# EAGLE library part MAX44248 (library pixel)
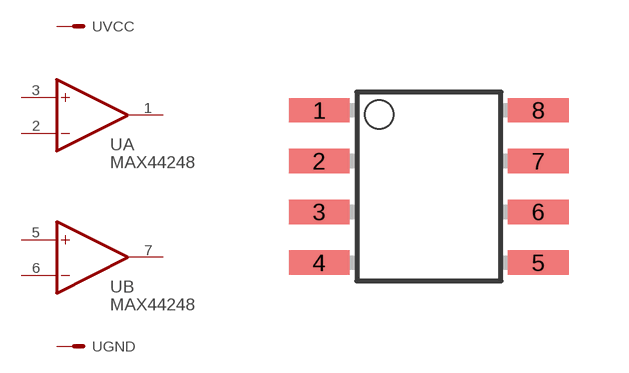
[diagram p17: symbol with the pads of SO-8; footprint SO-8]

Designator prefix -; gates A=OPAMP B=OPAMP VCC=M GND=M

## MAX44248  [SO-8]
1  A:OUT  out
2  A:-IN  in
3  A:+IN  in
4  GND:S  pas
5  B:+IN  in
6  B:-IN  in
7  B:OUT  out
8  VCC:S  pas

## Footprint SO-8 (pad centres in mm)
SO 8 small outline
smd 1.524 x 0.61: 1 -2.743,1.905; 2 -2.743,0.635; 3 -2.743,-0.635; 4 -2.743,-1.905; 5 2.743,-1.905; 6 2.743,-0.635; 7 2.743,0.635; 8 2.743,1.905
